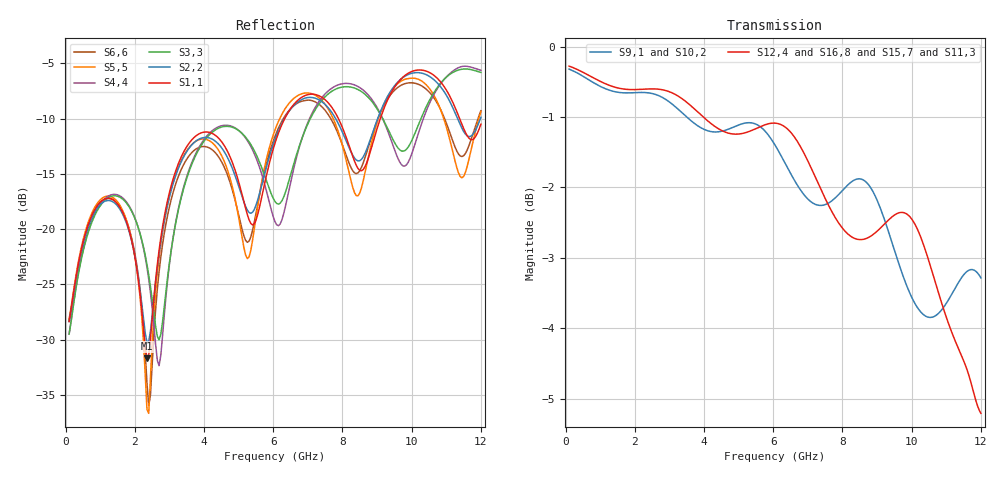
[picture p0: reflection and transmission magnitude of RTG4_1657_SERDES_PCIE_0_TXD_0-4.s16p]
! RTG4 1657 S-parameter file
! Microsemi Corporation (c) 2019
!Initial ver: Jul 30, 2019
! Port::PIN_NAME::NET_NAME::S-parameter ports::PORT SIDE
! Port1:--:SERDES_PCIE_0_TXD0_N_DIE::1::DIE
! Port2:--:SERDES_PCIE_0_TXD0_P_DIE::2::DIE
! Port3:AT3:SERDES_PCIE_0_TXD0_N_BGA::3::BGA
! Port4:AU3:SERDES_PCIE_0_TXD0_P_BGA::4::BGA
! Port5:--:SERDES_PCIE_0_TXD1_N_DIE::5::DIE
! Port6:--:SERDES_PCIE_0_TXD1_P_DIE::6::DIE
! Port7:AT5:SERDES_PCIE_0_TXD1_N_BGA::7::BGA
! Port8:AU5:SERDES_PCIE_0_TXD1_P_BGA::8::BGA
! Port9:--:SERDES_PCIE_0_TXD2_N_DIE::9::DIE
! Port10:--:SERDES_PCIE_0_TXD2_P_DIE::10::DIE
! Port11:AV6:SERDES_PCIE_0_TXD2_N_BGA::11::BGA
! Port12:AW6:SERDES_PCIE_0_TXD2_P_BGA::12::BGA
! Port13:--:SERDES_PCIE_0_TXD3_N_DIE::13::DIE
! Port14:--:SERDES_PCIE_0_TXD3_P_DIE::14::DIE
! Port15:AV8:SERDES_PCIE_0_TXD3_N_BGA::15::BGA
! Port16:AW8:SERDES_PCIE_0_TXD3_P_BGA::16::BGA
!TouchstoneFormatFlag = 1
! GNDNET
! NETSLIST
! User Comments:
! Touchstone file exported from HFSS 2018.2.0
!  File:  //LSI_Z840_SIM_PC/Simulation_Data/MASUMISU/Microsemi_190710/YBD197_150320_NETCHANGE_SERDES_PCIE_0_TXD.aedt
!  Generated:  9:24:34 ??  7 16, 2019
!  Design:  HFSSModel1
!  Project:  YBD197_150320_NETCHANGE_SERDES_PCIE_0_TXD
!  Setup:  Setup1
!  Solution:  Sweep
! Terminal data exported
! Port[1] = SERDES_PCIE_0_TXD0_N_DIE
! Port[2] = SERDES_PCIE_0_TXD0_P_DIE
! Port[3] = SERDES_PCIE_0_TXD1_N_DIE
! Port[4] = SERDES_PCIE_0_TXD1_P_DIE
! Port[5] = SERDES_PCIE_0_TXD2_N_DIE
! Port[6] = SERDES_PCIE_0_TXD2_P_DIE
! Port[7] = SERDES_PCIE_0_TXD3_N_DIE
! Port[8] = SERDES_PCIE_0_TXD3_P_DIE
! Port[9] = SERDES_PCIE_0_TXD0_N_BGA
! Port[10] = SERDES_PCIE_0_TXD0_P_BGA
! Port[11] = SERDES_PCIE_0_TXD1_N_BGA
! Port[12] = SERDES_PCIE_0_TXD1_P_BGA
! Port[13] = SERDES_PCIE_0_TXD2_N_BGA
! Port[14] = SERDES_PCIE_0_TXD2_P_BGA
! Port[15] = SERDES_PCIE_0_TXD3_N_BGA
! Port[16] = SERDES_PCIE_0_TXD3_P_BGA
# GHZ S DB R 50.000000
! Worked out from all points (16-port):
!   239 points, 100 MHz to 12 GHz, reference 50 ohm
!   strongest paths, dB at 100 MHz, 3.05 GHz, 6.05 GHz, 9.05 GHz, 12 GHz:
!     S12,4: -0.3, -0.7, -1.1, -2.6, -5.2
!     S16,8: -0.3, -0.7, -1.2, -2.4, -4.3
!     S15,7: -0.3, -0.7, -1.2, -2.4, -4.4
!     S11,3: -0.3, -0.7, -1.2, -2.6, -4.9
!     S9,1: -0.3, -0.8, -1.4, -2.2, -3.3
!     S10,2: -0.3, -0.8, -1.4, -2.4, -3.5
!   lowest |S11| = -31.7 dB at 2.35 GHz (marker M1), VSWR 1.05, Z = 51.6 + j2.13 ohm
!   |S11| at or under -10 dB: start of sweep to 6.331 GHz; 7.882 GHz to 9.094 GHz (1.212 GHz wide, 14.3 % of centre); 11.39 GHz to end of sweep
